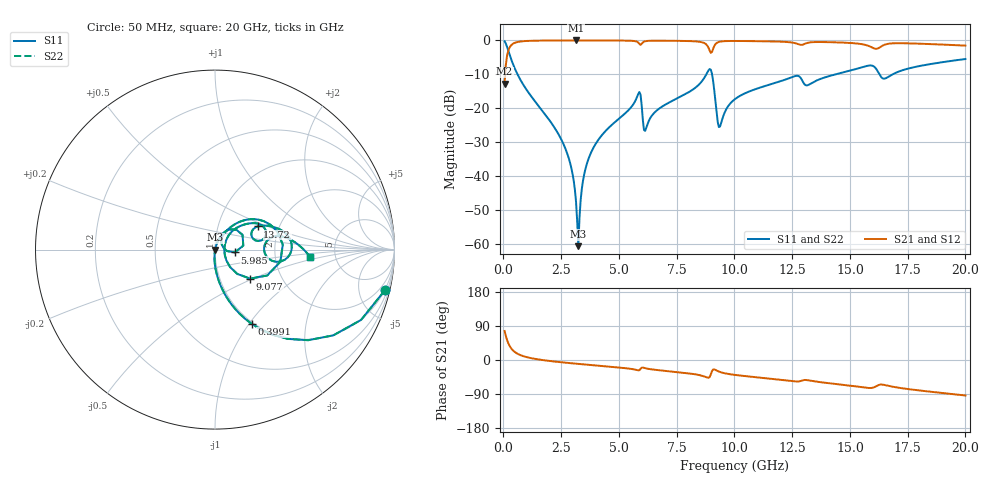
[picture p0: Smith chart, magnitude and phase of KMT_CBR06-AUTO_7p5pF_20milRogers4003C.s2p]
! Data measured by Modelithics Inc. support@modelithics.com 813-866-6335
! KEMET CBR06-AUTO 7.5pF, Pad Width= 0.851mm, Pad Length= 0.64mm, Pad Gap= 0.62mm, 20mil Rogers 4003C substrate Data, January 2022
# hz S ma R 50
! 2 Port Network Data from SP1.SP block
! freq  magS11  angS11  magS21  angS21  magS12  angS12  magS22  angS22
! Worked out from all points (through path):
!   401 points, 50 MHz to 20 GHz, reference 50 ohm
!   highest |S21| = -0.01 dB at 3.142 GHz (marker M1); lowest = -12.7 dB at 50 MHz (marker M2)
!   group delay of S21, straight-line fit = 14.3 ps
!   lowest |S11| = -60.6 dB at 3.242 GHz (marker M3), VSWR 1.00, Z = 50.1 - j0.00177 ohm
!   |S11| at or under -10 dB: 610 MHz to 8.782 GHz (8.172 GHz wide, 174 % of centre); 9.033 GHz to 14.37 GHz (5.34 GHz wide, 45.6 % of centre); 16.28 GHz to 16.85 GHz (570.6 MHz wide, 3.45 % of centre)
!   |S22| runs from -60.6 to -0.2 dB; largest |S21 - S12| = 0
!   S11 on the Smith chart (normalised r, x): 50 MHz: 0.98, -8.32; 399.1 MHz: 0.98, -1.03; 5.985 GHz: 1.25, -0.04; 9.077 GHz: 1.39, -0.48; 13.72 GHz: 1.55, +0.43; 20 GHz: 3.23, -0.37
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5e7  0.9729 -13.5  0.2311 76.5  0.2311 76.5  0.9729 -13.5
3.99125e8  0.461 -63.8  0.8868 26.2  0.8868 26.2  0.461 -63.8
2.593625e9  0.03005 -94.9  0.9986 -6.5  0.9986 -6.5  0.03005 -94.9
2.94275e9  0.01304 -94.8  0.9989 -8.6  0.9989 -8.6  0.01304 -94.8
3.14225e9  0.004219 -87.3  0.999 -9.8  0.999 -9.8  0.004219 -87.3
3.242e9  0.0009336 -1.1  0.999 -10.3  0.999 -10.3  0.0009336 -1.1
3.391625e9  0.006447 70.4  0.9989 -11.1  0.9989 -11.1  0.006447 70.4
3.641e9  0.01641 74.0  0.9987 -12.5  0.9987 -12.5  0.01641 74.0
4.13975e9  0.03561 73.0  0.9981 -15.2  0.9981 -15.2  0.03561 73.0
5.8355e9  0.1627 42.2  0.9309 -27.2  0.9309 -27.2  0.1627 42.2
5.985125e9  0.1107 -8.1  0.8913 -20.3  0.8913 -20.3  0.1107 -8.1
6.184625e9  0.05185 46.1  0.9795 -22.3  0.9795 -22.3  0.05185 46.1
6.73325e9  0.09868 60.6  0.9907 -27.0  0.9907 -27.0  0.09868 60.6
8.678375e9  0.2752 38.1  0.92 -43.1  0.92 -43.1  0.2752 38.1
9.077375e9  0.254 -39.6  0.7519 -24.9  0.7519 -24.9  0.254 -39.6
9.376625e9  0.05404 12.1  0.9599 -31.7  0.9599 -31.7  0.05404 12.1
1.0025e10  0.1368 46.9  0.9815 -39.4  0.9815 -39.4  0.1368 46.9
1.336662e10  0.2377 27.6  0.9422 -55.4  0.9422 -55.4  0.2377 27.6
1.371575e10  0.2704 28.4  0.9477 -58.4  0.9477 -58.4  0.2704 28.4
1.586038e10  0.428 3.7  0.8165 -73.9  0.8165 -73.9  0.428 3.7
1.670825e10  0.2969 10.0  0.8976 -68.7  0.8976 -68.7  0.2969 10.0
2e10  0.5323 -4.5  0.8382 -93.6  0.8382 -93.6  0.5323 -4.5
